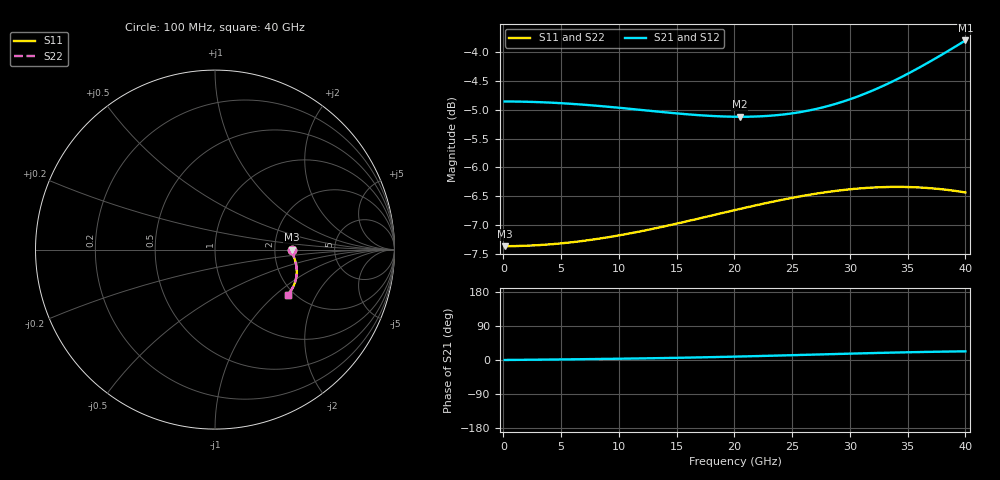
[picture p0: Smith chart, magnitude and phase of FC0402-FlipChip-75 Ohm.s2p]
!Vishay Thin-Film
!FC Family
!Case Size 0402
!Assembly Style Flip-Chip
!10/21/2015
!thinfilm@vishay.com
# GHz S MA R 50
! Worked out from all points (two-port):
!   101 points, 100 MHz to 40 GHz, reference 50 ohm
!   highest |S21| = -3.81 dB at 40 GHz (marker M1); lowest = -5.1 dB at 20.45 GHz (marker M2)
!   |S21| within 3 dB of the highest: start of sweep to end of sweep
!   lowest |S11| = -7.4 dB at 100 MHz (marker M3), VSWR 2.50, Z = 125 - j0.0903 ohm
!   |S11| at or under -10 dB: nowhere
!   |S22| runs from -7.4 to -6.3 dB; largest |S21 - S12| = 0
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0.1  0.4286 -0.0  0.5714 0.0  0.5714 0.0  0.4286 -0.0
3.292  0.4296 -1.3  0.5706 1.0  0.5706 1.0  0.4296 -1.3
6.883  0.4331 -2.8  0.5679 2.2  0.5679 2.2  0.4331 -2.8
10.474  0.4387 -4.6  0.5638 3.6  0.5638 3.6  0.4387 -4.6
13.666  0.4452 -6.3  0.5597 5.0  0.5597 5.0  0.4452 -6.3
15.262  0.4488 -7.3  0.5578 5.9  0.5578 5.9  0.4488 -7.3
16.858  0.4526 -8.4  0.5562 6.8  0.5562 6.8  0.4526 -8.4
18.454  0.4565 -9.5  0.555 7.8  0.555 7.8  0.4565 -9.5
20.05  0.4605 -10.8  0.5544 8.9  0.5544 8.9  0.4605 -10.8
20.449  0.4614 -11.1  0.5543 9.2  0.5543 9.2  0.4614 -11.1
22.045  0.4653 -12.4  0.5547 10.4  0.5547 10.4  0.4653 -12.4
23.641  0.4689 -13.8  0.5561 11.6  0.5561 11.6  0.4689 -13.8
25.237  0.4723 -15.3  0.5586 12.9  0.5586 12.9  0.4723 -15.3
26.833  0.4753 -16.9  0.5623 14.2  0.5623 14.2  0.4753 -16.9
28.828  0.4784 -18.9  0.569 15.8  0.569 15.8  0.4784 -18.9
30.424  0.4803 -20.6  0.576 17.1  0.576 17.1  0.4803 -20.6
32.02  0.4816 -22.4  0.5844 18.3  0.5844 18.3  0.4816 -22.4
33.616  0.4822 -24.2  0.5942 19.4  0.5942 19.4  0.4822 -24.2
35.212  0.482 -26.1  0.6053 20.5  0.6053 20.5  0.482 -26.1
36.808  0.4811 -27.9  0.6176 21.4  0.6176 21.4  0.4811 -27.9
38.404  0.4794 -29.8  0.631 22.2  0.631 22.2  0.4794 -29.8
40  0.4769 -31.7  0.6452 22.9  0.6452 22.9  0.4769 -31.7
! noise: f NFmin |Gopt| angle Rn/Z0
0.1  -2.893e-15  1  -2.537e-17  1.5
4.489  2.893e-15  1  1.014e-16  1.509
8.878  1.929e-15  1  -8.538e-07  1.531
13.27  1.425e-07  1  -4.067e-15  1.557
17.66  1.929e-15  1  -1.207e-06  1.571
22.05  -9.643e-16  1  -8.538e-07  1.546
26.43  -2.411e-15  1  -2.594e-15  1.459
30.82  1.192e-07  1  0  1.302
35.21  0  1  -3.963e-15  1.095
40  7.835e-08  1  2.231e-15  0.8561
